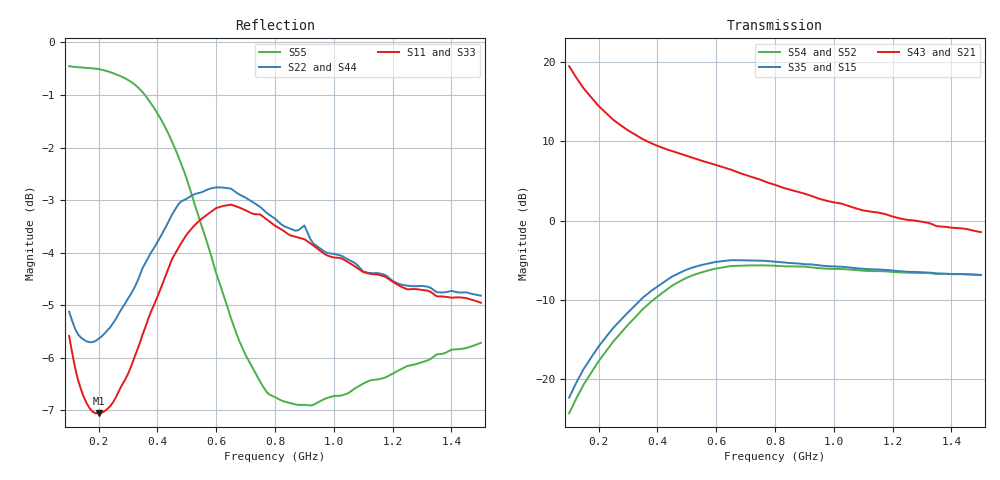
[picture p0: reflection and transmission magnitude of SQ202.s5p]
!  POLYFET RF DEVICES
!  S PARAMETERS FOR
!  SQ202 (PER SIDE)
!  VDS=28, IDQ=400MA
! Date: Thu Sep 24 14:52:01 1998
!AWR Design Environment (2053) Wed Feb 04 15:57:40 2004
!freq-unit  param-type  data-format  keyword  impedance-ohms
# MHz  S  MA  R  50
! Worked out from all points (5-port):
!   141 points, 100 MHz to 1.5 GHz, reference 50 ohm
!   strongest paths, dB at 100 MHz, 450 MHz, 800 MHz, 1.15 GHz, 1.5 GHz:
!     S43: 19.4, 8.7, 4.5, 1.0, -1.5
!     S21: 19.4, 8.7, 4.5, 1.0, -1.5
!     S35: -22.3, -7.0, -5.2, -6.1, -6.9
!     S15: -22.3, -7.0, -5.2, -6.1, -6.9
!     S54: -24.3, -8.2, -5.7, -6.4, -6.8
!     S52: -24.3, -8.2, -5.7, -6.4, -6.8
!   lowest |S11| = -7.1 dB at 200 MHz (marker M1), VSWR 2.60, Z = 51.9 - j50.4 ohm
!   |S11| at or under -10 dB: nowhere
